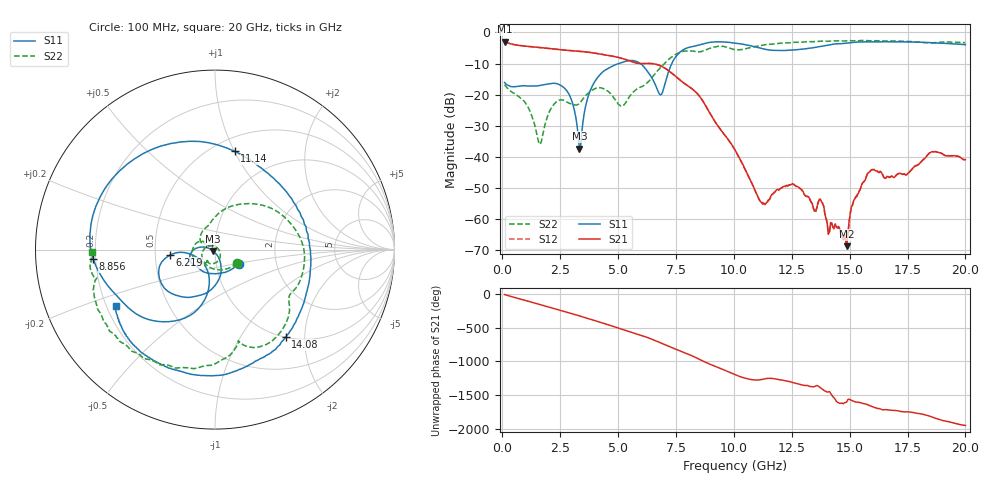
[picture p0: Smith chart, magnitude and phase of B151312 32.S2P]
!  2-Port S-parameters saved by WinCal
! VAR MeasName=S-Parameters (CALIBRATED_DATA) read from VNA (N5244A)
! VAR MeasDate=12/8/2015 5:45:58 PM
! VAR NAME=B151312 32
! VAR FILENAME=B151312 32.S2P
! VAR DATE=12/8/2015 5:45:58 PM
! VAR PHYS_PORTS=1,2
# Hz S DB R 50
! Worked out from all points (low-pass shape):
!   401 points, 100 MHz to 20 GHz, reference 50 ohm
!   highest |S21| = -2.99 dB at 100 MHz (marker M1); lowest = -68.6 dB at 14.88 GHz (marker M2)
!   |S21| within 3 dB of the highest: start of sweep to 3.227 GHz
!   lowest |S11| = -37.3 dB at 3.334 GHz (marker M3), VSWR 1.03, Z = 48.8 - j0.691 ohm
!   |S11| at or under -10 dB: start of sweep to 5.029 GHz; 5.963 GHz to 7.32 GHz (1.357 GHz wide, 20.4 % of centre)
!   |S22| runs from -35.9 to -2.6 dB; largest |S21 - S12| = 0.0013
!   S11 on the Smith chart (normalised r, x): 100 MHz: 1.30, -0.21; 6.219 GHz: 0.60, -0.04; 8.856 GHz: 0.19, -0.04; 11.14 GHz: 0.63, +1.00; 14.08 GHz: 1.01, -1.61; 20 GHz: 0.24, -0.25
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1e8  -16.08 -29.8  -2.99 -13.4  -2.99 -13.4  -16.77 -31.1
8.96e8  -17.11 -117.8  -4.33 -91.0  -4.33 -91.0  -21.74 -152.5
1.74175e9  -16.86 -141.9  -4.94 -171.9  -4.95 -172.0  -33.00 -4.7
2.7865e9  -18.74 179.1  -5.74 86.8  -5.74 86.7  -22.39 -125.0
3.33375e9  -37.28 -148.9  -6.06 31.8  -6.06 31.8  -22.76 -123.3
3.43325e9  -32.16 -75.8  -6.13 21.6  -6.13 21.6  -21.85 -123.7
3.7815e9  -18.98 -72.1  -6.43 -14.7  -6.42 -14.7  -19.04 -135.5
4.478e9  -11.94 -103.2  -7.27 -88.8  -7.26 -88.7  -18.46 170.6
5.274e9  -9.39 -132.6  -8.60 -177.1  -8.58 -177.1  -23.07 154.4
6.21925e9  -12.00 -173.1  -9.97 79.2  -9.98 79.2  -16.46 100.3
6.7665e9  -19.52 -152.3  -10.52 4.9  -10.53 4.9  -11.84 70.0
7.71175e9  -6.12 -125.6  -15.55 -128.0  -15.50 -128.1  -6.26 4.7
8.856e9  -3.34 -175.5  -24.52 56.2  -24.48 55.8  -5.41 -39.3
1.005e10  -3.41 131.3  -37.75 -114.2  -37.77 -114.4  -5.54 -75.6
1.11445e10  -5.06 78.6  -54.28 172.1  -54.43 172.0  -4.27 -85.7
1.248775e10  -5.63 13.9  -48.81 135.8  -48.97 136.9  -3.25 -106.9
1.338325e10  -4.97 -25.7  -54.93 69.4  -54.86 70.2  -2.99 -117.7
1.407975e10  -4.08 -50.9  -64.83 -8.2  -64.26 -11.5  -2.83 -126.4
1.487575e10  -3.43 -74.5  -68.64 -156.7  -68.50 -143.9  -2.69 -135.2
1.5821e10  -3.02 -98.2  -45.01 155.4  -44.82 155.7  -2.66 -144.9
1.67165e10  -3.03 -113.9  -46.57 84.3  -46.41 84.5  -2.70 -153.0
2e10  -3.95 -150.5  -40.85 -142.5  -40.86 -143.9  -3.29 -178.9
